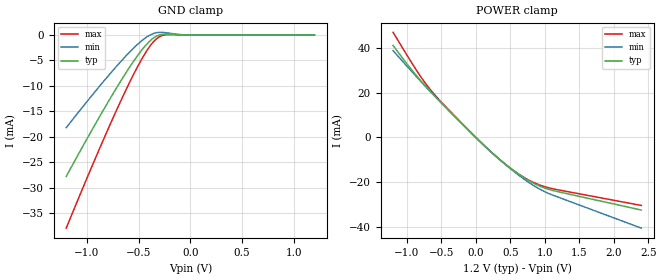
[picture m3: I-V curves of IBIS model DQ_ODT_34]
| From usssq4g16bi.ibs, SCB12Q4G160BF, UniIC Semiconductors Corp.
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|   Model DQ_ODT_34
[Model] DQ_ODT_34
Model_type Input
Polarity   Non-Inverting
Enable   Active-High
Vinl =  8.300E-01
Vinh =  9.700E-01
C_comp   7.640E-13   7.515E-13   7.899E-13
C_comp_power_clamp   1.804E-13   1.542E-13   2.173E-13
C_comp_gnd_clamp   5.836E-13   5.726E-13   5.973E-13
[Model Spec]
Vinh   9.700E-01   9.250E-01   1.015E+00
Vinl   8.300E-01   7.850E-01   8.750E-01
[Temperature Range]   45.000   95.000   -40.000
[Voltage Range]   1.200E+00   1.140E+00   1.260E+00
[C Comp Corner]
C_comp_power_clamp   1.804E-13   1.542E-13   2.173E-13
C_comp_gnd_clamp   5.836E-13   5.973E-13   5.726E-13
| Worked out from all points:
|   GND clamp passes 1 mA (typ) near -0.38 V on its own axis
|   POWER clamp passes 1 mA (typ) near -0.03 V on its own axis
[GND_clamp]
|Voltage   I(typ)   I(min)   I(max)
-1.2V     -27.79mA   -18.22mA   -37.96mA
-875mV    -15.96mA   -9.999mA   -22.19mA
-750mV    -11.63mA   -7mA       -16.42mA
-625mV    -7.509mA   -4.17mA    -10.9mA
-525mV    -4.476mA   -2.121mA   -6.807mA
-450mV    -2.469mA   -812.5uA   -4.049mA
-375mV    -882.6uA   133.3uA    -1.777mA
-325mV    -202.5uA   453.1uA    -711uA
-275mV    112.6uA    510.7uA    -122.8uA
-200mV    151uA      340.7uA    80.06uA
-25mV     0A         0A         0A
1.2V      0A         0A         0A
[POWER_clamp]
|Voltage   I(typ)   I(min)   I(max)
-1.2V     41.15mA    38.85mA    47.03mA
-1V       32.96mA    31.91mA    36.88mA
-825mV    26.34mA    25.96mA    28.37mA
-700mV    22.02mA    21.8mA     22.97mA
-600mV    18.75mA    18.57mA    19.2mA
-300mV    9.243mA    9.156mA    9.395mA
125mV     -3.71mA    -3.691mA   -3.77mA
350mV     -9.936mA   -10.01mA   -10.02mA
575mV     -15.42mA   -15.77mA   -15.4mA
825mV     -20.27mA   -21.26mA   -19.95mA
1.05V     -23.13mA   -24.98mA   -22.46mA
2.4V      -32.46mA   -40.56mA   -30.41mA
